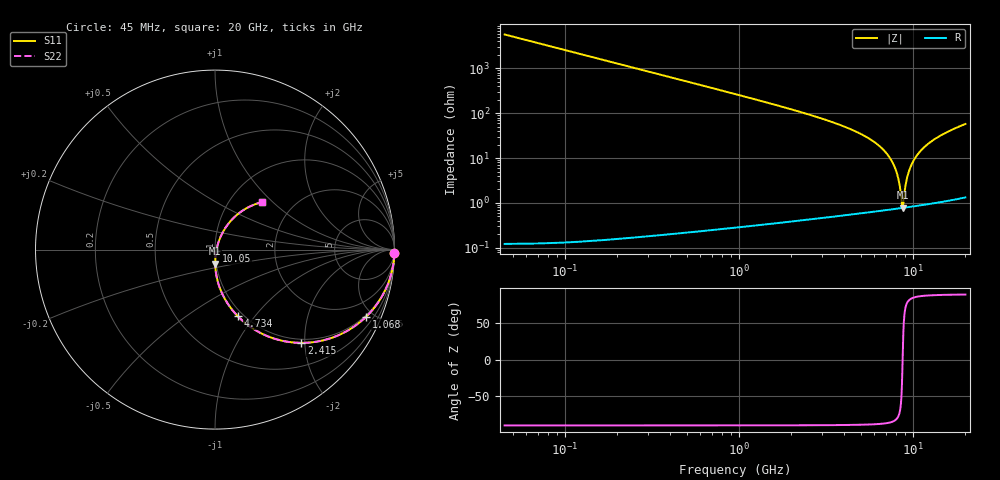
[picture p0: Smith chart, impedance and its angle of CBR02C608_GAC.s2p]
! S-parameter model data by Modelithics Inc.  support@modelithics.com 813-866-6335  Tampa FL USA
! S-Parameter data specifications:
! Substrate: 20-mil Rogers 4350B, substrate thickness, H=0.508mm, Dielectric constant, Er=3.75
! PCB Mounting Pad Footprint: Pad width, PadW=0.32mm , Pad length, PadL=0.37mm , Pad gap, PadG (edge-to-edge)=0.19mm , Reference planes=0.93mm apart
#  GHz  S  MA  R 50
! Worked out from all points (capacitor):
!   801 points, 45 MHz to 20 GHz, reference 50 ohm
!   read as one part in series: C = 619 fF near 144.8 MHz
!   lowest |Z| = 774 mohm at 8.725 GHz (marker M1)
!   series resonance near 8.714 GHz, so ESL is about 540 pH
!   S11 on the Smith chart (normalised r, x): 45 MHz: open; 1.068 GHz: 0.92, -4.55; 2.415 GHz: 0.92, -1.93; 4.734 GHz: 0.94, -0.82; 10.05 GHz: 1.01, -0.02; 20 GHz: 1.41, +0.87
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0.045  0.9998 -1.1  0.0175 88.9  0.0175 88.9  0.9998 -1.1
0.219606  0.9964 -5.1  0.08514 84.9  0.08514 84.9  0.9964 -5.1
0.369269  0.9898 -8.6  0.1423 81.4  0.1423 81.4  0.9898 -8.6
0.668594  0.9674 -15.3  0.2526 74.6  0.2526 74.6  0.9674 -15.3
1.067694  0.9216 -23.9  0.3869 66.0  0.3869 66.0  0.9216 -23.9
1.691288  0.8275 -35.8  0.5594 54.1  0.5594 54.1  0.8275 -35.8
2.414656  0.7079 -47.2  0.7034 42.5  0.7034 42.5  0.7079 -47.2
3.387462  0.5587 -59.2  0.8253 30.4  0.8253 30.4  0.5587 -59.2
4.734425  0.3917 -71.2  0.9149 18.1  0.9149 18.1  0.3917 -71.2
6.704981  0.2131 -83.0  0.9704 5.3  0.9704 5.3  0.2131 -83.0
8.725425  0.0788 -89.1  0.9892 -4.7  0.9892 -4.7  0.0788 -89.1
9.523625  0.03456 -84.7  0.9913 -8.1  0.9913 -8.1  0.03456 -84.7
9.773062  0.0219 -77.4  0.9915 -9.1  0.9915 -9.1  0.0219 -77.4
10.0225  0.01104 -52.0  0.9916 -10.1  0.9916 -10.1  0.01104 -52.0
10.04744  0.01024 -46.7  0.9916 -10.2  0.9916 -10.2  0.01024 -46.7
10.22205  0.00877 7.7  0.9915 -10.9  0.9915 -10.9  0.00877 7.7
10.72092  0.02875 59.9  0.9909 -12.8  0.9909 -12.8  0.02875 59.9
11.34452  0.05758 66.0  0.9893 -15.2  0.9893 -15.2  0.05758 66.0
12.19261  0.09528 66.2  0.9861 -18.2  0.9861 -18.2  0.09528 66.2
13.36496  0.1442 63.9  0.9797 -22.3  0.9797 -22.3  0.1442 63.9
16.68248  0.2674 54.6  0.9523 -33.0  0.9523 -33.0  0.2674 54.6
20  0.3744 45.1  0.9146 -43.0  0.9146 -43.0  0.3744 45.1
